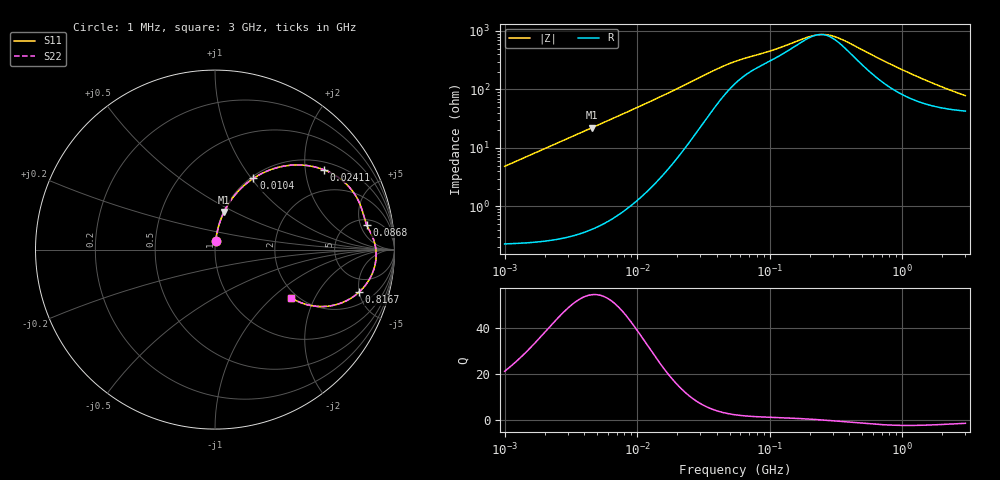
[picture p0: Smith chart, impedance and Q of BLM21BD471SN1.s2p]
! BLM21BD471SN1
# Hz S RI R 50
!Freq.(Hz) S11(Real) S11(Imag) S21(Real) S21(Imag) S12(Real) S12(Imag) S22(Real) S22(Imag)
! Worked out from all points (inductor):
!   401 points, 1 MHz to 3 GHz, reference 50 ohm
!   read as one part in series: L = 770 nH near 1.041 MHz
!   highest Q = 54.6 at 4.578 MHz (marker M1), where L = 772 nH
!   self-resonance near 237.2 MHz
!   S11 on the Smith chart (normalised r, x): 1 MHz: 1.00, +0.10; 10.4 MHz: 1.03, +1.02; 24.11 MHz: 1.23, +2.52; 86.8 MHz: 6.15, +6.39; 816.7 MHz: 3.14, -4.96; 3 GHz: 1.85, -1.32
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1000000  0.0046 0.048  0.9954 -0.048  0.9954 -0.048  0.0046 0.048
2055611  0.0123 0.098  0.9877 -0.098  0.9877 -0.098  0.0123 0.098
3823119  0.0363 0.178  0.9637 -0.178  0.9637 -0.178  0.0363 0.178
4577760  0.0505 0.21  0.9495 -0.21  0.9495 -0.21  0.0505 0.21
7110411  0.1122 0.3056  0.8878 -0.3056  0.8878 -0.3056  0.1122 0.3056
1.040059e7  0.2137 0.3969  0.7863 -0.3969  0.7863 -0.3969  0.2137 0.3969
1.461624e7  0.3537 0.4587  0.6463 -0.4587  0.6463 -0.4587  0.3537 0.4587
1.896016e7  0.4844 0.4711  0.5156 -0.4711  0.5156 -0.4711  0.4844 0.4711
2.41077e7  0.6055 0.4452  0.3945 -0.4452  0.3945 -0.4452  0.6055 0.4452
3.597591e7  0.7567 0.3382  0.2433 -0.3382  0.2433 -0.3382  0.7567 0.3382
5.477226e7  0.8203 0.2176  0.1797 -0.2176  0.1797 -0.2176  0.8203 0.2176
8.679508e7  0.8445 0.1391  0.1555 -0.1391  0.1555 -0.1391  0.8445 0.1391
2.094008e8  0.8934 0.02  0.1066 -0.02  0.1066 -0.02  0.8934 0.02
2.558035e8  0.8976 -0.0125  0.1024 0.0125  0.1024 0.0125  0.8976 -0.0125
3.124888e8  0.8973 -0.0471  0.1027 0.0471  0.1027 0.0471  0.8973 -0.0471
5.154121e8  0.8716 -0.1436  0.1284 0.1436  0.1284 0.1436  0.8716 -0.1436
8.005644e8  0.8058 -0.2339  0.1942 0.2339  0.1942 0.2339  0.8058 -0.2339
8.167498e8  0.8016 -0.2378  0.1984 0.2378  0.1984 0.2378  0.8016 -0.2378
1.147801e9  0.7139 -0.2933  0.2861 0.2933  0.2861 0.2933  0.7139 -0.2933
1.54974e9  0.6177 -0.3165  0.3823 0.3165  0.3823 0.3165  0.6177 -0.3165
2.092429e9  0.5198 -0.3087  0.4802 0.3087  0.4802 0.3087  0.5198 -0.3087
3e9  0.4221 -0.2669  0.5779 0.2669  0.5779 0.2669  0.4221 -0.2669
